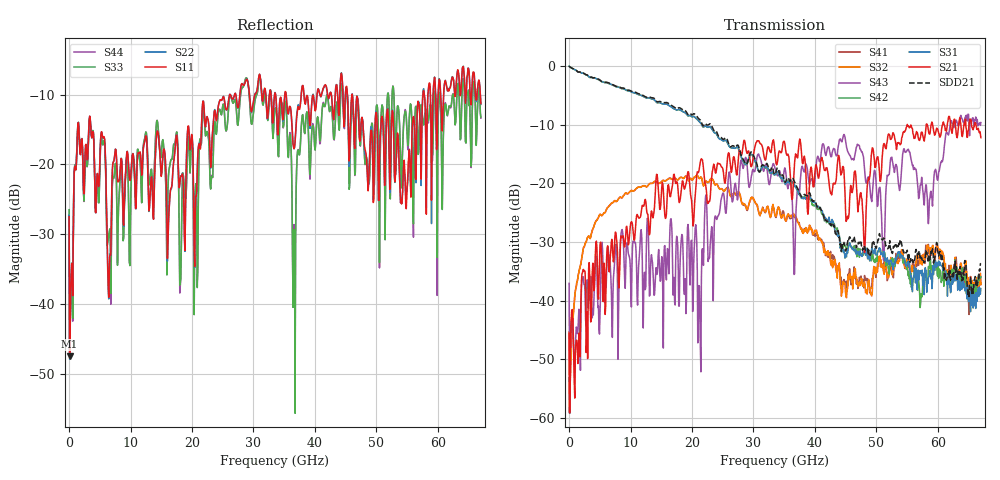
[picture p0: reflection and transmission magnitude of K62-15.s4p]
!Agilent Technologies,N5247A,US50470101,A.10.25.02
!Agilent N5247A: A.10.25.02
!Date: Tuesday, May 12, 2015 13:40:47
!Correction: Sdd11(Full 4 Port(1,2,3,4))
!Sdc11(Full 4 Port(1,2,3,4))
!Sdd12(Full 4 Port(1,2,3,4))
!Sdc12(Full 4 Port(1,2,3,4))
!Scd11(Full 4 Port(1,2,3,4))
!Scc11(Full 4 Port(1,2,3,4))
!Scd12(Full 4 Port(1,2,3,4))
!Scc12(Full 4 Port(1,2,3,4))
!Sdd21(Full 4 Port(1,2,3,4))
!Sdc21(Full 4 Port(1,2,3,4))
!Sdd22(Full 4 Port(1,2,3,4))
!Sdc22(Full 4 Port(1,2,3,4))
!Scd21(Full 4 Port(1,2,3,4))
!Scc21(Full 4 Port(1,2,3,4))
!Scd22(Full 4 Port(1,2,3,4))
!Scc22(Full 4 Port(1,2,3,4))
!Balanced Topology: BBAL
!S4P File: Measurements: <Sdd11,Sdc11,Sdd12,Sdc12>,
!<Scd11,Scc11,Scd12,Scc12>,
!<Sdd21,Sdc21,Sdd22,Sdc22>,
!<Scd21,Scc21,Scd22,Scc22>:
# Hz S  dB  R 50
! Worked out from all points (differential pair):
!   801 points, 10 MHz to 67 GHz, reference 50 ohm
!   strongest paths, dB at 10 MHz, 16.76 GHz, 33.51 GHz, 50.25 GHz, 67 GHz:
!     S21: -45.5, -20.7, -14.9, -15.5, -12.2
!     S31: 0.0, -7.1, -18.5, -31.7, -37.9
!     S42: 0.0, -7.1, -18.5, -31.5, -36.0
!     S43: -37.0, -28.8, -17.4, -23.6, -9.6
!     S32: -45.3, -19.3, -25.5, -34.2, -37.3
!     S41: -53.2, -19.3, -25.3, -33.8, -37.2
!   taken as a pair (ports 1,2 in; 3,4 out), SDD21 dB: 0.0, -6.8, -18.5, -29.6, -33.6
!   lowest |S11| = -47.5 dB at 93.74 MHz (marker M1), VSWR 1.01, Z = 50.2 - j0.389 ohm
!   |S11| at or under -10 dB: start of sweep to 26.12 GHz; 35.31 GHz to 37.77 GHz (2.457 GHz wide, 6.72 % of centre); 46.08 GHz to 57.58 GHz (11.5 GHz wide, 22.2 % of centre)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
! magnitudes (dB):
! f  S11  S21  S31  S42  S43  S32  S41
! 10 MHz  -27.5  -45.5  0.0  0.0  -37.0  -45.3  -53.2
! 93.74 MHz  -47.5  -59.1  -0.1  -0.1  -59.2  -58.4  -59.2
! 3.527 GHz  -14.6  -43.7  -1.9  -1.9  -35.9  -29.1  -29.1
! 6.458 GHz  -39.0  -34.8  -3.0  -3.0  -32.1  -23.9  -23.9
! 16.26 GHz  -26.8  -20.8  -6.7  -6.7  -35.4  -19.2  -19.2
! 28.73 GHz  -8.0  -13.8  -16.8  -16.8  -15.6  -23.8  -24.0
! 67 GHz  -11.3  -12.2  -37.9  -36.0  -9.6  -37.3  -37.2
